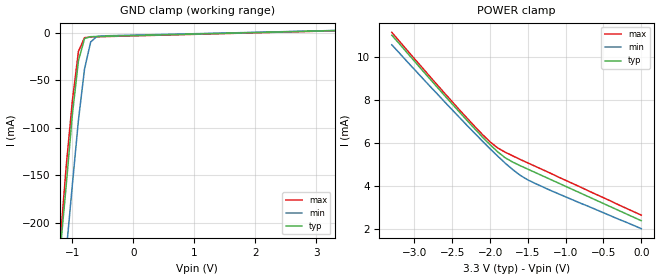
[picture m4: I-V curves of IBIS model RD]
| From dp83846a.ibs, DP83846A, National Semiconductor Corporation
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|   Model RD
[Model]   RD
Model_type   Input
Polarity   Non-Inverting
Enable   Active-High
Vinl =   0.80V
Vinh =   2.00V
Vmeas =   1.50V
Cref =  20.00pF
Rref = 100.00k
C_comp   5.00pF   5.00pF   5.00pF
[Temperature Range]   25.00   0.14k   0.000
[Voltage Range]   3.30V   3.00V   3.60V
[GND_clamp]
| voltage   I(typ)   I(min)   I(max)
-3.3V     -1.98A     -2.04A     -1.96A
-1.2V     -230mA     -310mA     -220mA
-1.1V     -160mA     -230mA     -140mA
-1V       -86.21mA   -160mA     -71.7mA
-900mV    -29.33mA   -91.84mA   -19.52mA
-800mV    -6.07mA    -37.93mA   -5.11mA
-700mV    -4.08mA    -9.68mA    -4.36mA
-600mV    -3.86mA    -3.9mA     -4.19mA
3.3V      2.37mA     2.44mA     2.14mA
[POWER_clamp]
| voltage   I(typ)   I(min)   I(max)
-3.3V     11.01mA    10.56mA    11.14mA
-2.6V     8.19mA     7.9mA      8.3mA
-2.2V     6.64mA     6.43mA     6.75mA
-2V       5.91mA     5.72mA     6.04mA
-1.9V     5.58mA     5.38mA     5.76mA
-1.8V     5.3mA      5.05mA     5.56mA
-1.6V     4.93mA     4.48mA     5.22mA
-1.4V     4.61mA     4.1mA      4.9mA
0V        2.37mA     2mA        2.63mA
